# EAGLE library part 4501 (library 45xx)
NAND/NOR/OR
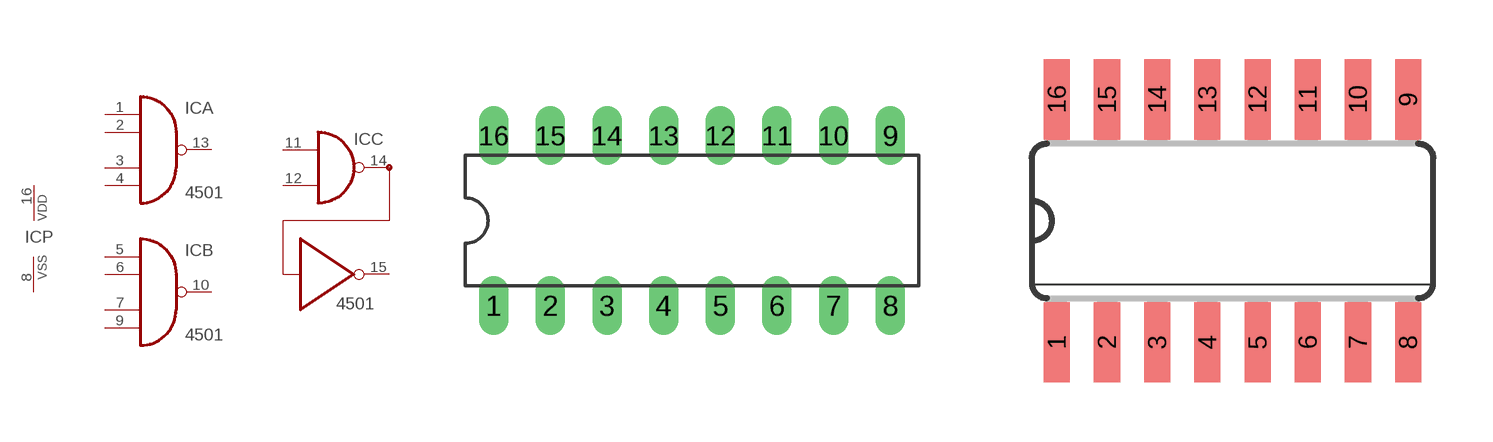
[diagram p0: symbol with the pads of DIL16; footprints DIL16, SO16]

Designator prefix IC; gates A=4501 B=4501 C=4501/A P=PWRN

## 4501N  [DIL16]
1  A:I0  in
2  A:I1  in
3  A:I2  in
4  A:I3  in
5  B:I0  in
6  B:I1  in
7  B:I2  in
8  P:VSS  pwr
9  B:I3  in
10  B:O  out
11  C:I0  in
12  C:I1  in
13  A:O  out
14  C:O1  out
15  C:O2  out
16  P:VDD  pwr

## 4501D  [SO16]
Pads as for DIL16

## Footprint DIL16 (pad centres in mm)
Dual In Line Package
drill 0.813 long: 1 -8.89,-3.81; 2 -6.35,-3.81; 3 -3.81,-3.81; 4 -1.27,-3.81; 5 1.27,-3.81; 6 3.81,-3.81; 7 6.35,-3.81; 8 8.89,-3.81; 9 8.89,3.81; 10 6.35,3.81; 11 3.81,3.81; 12 1.27,3.81; 13 -1.27,3.81; 14 -3.81,3.81; 15 -6.35,3.81; 16 -8.89,3.81

## Footprint SO16 (pad centres in mm)
Small Outline package 150 mil
smd 0.66 x 2.032: 1 -4.445,-3.073; 2 -3.175,-3.073; 3 -1.905,-3.073; 4 -0.635,-3.073; 5 0.635,-3.073; 6 1.905,-3.073; 7 3.175,-3.073; 8 4.445,-3.073; 9 4.445,3.073; 10 3.175,3.073; 11 1.905,3.073; 12 0.635,3.073; 13 -0.635,3.073; 14 -1.905,3.073; 15 -3.175,3.073; 16 -4.445,3.073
